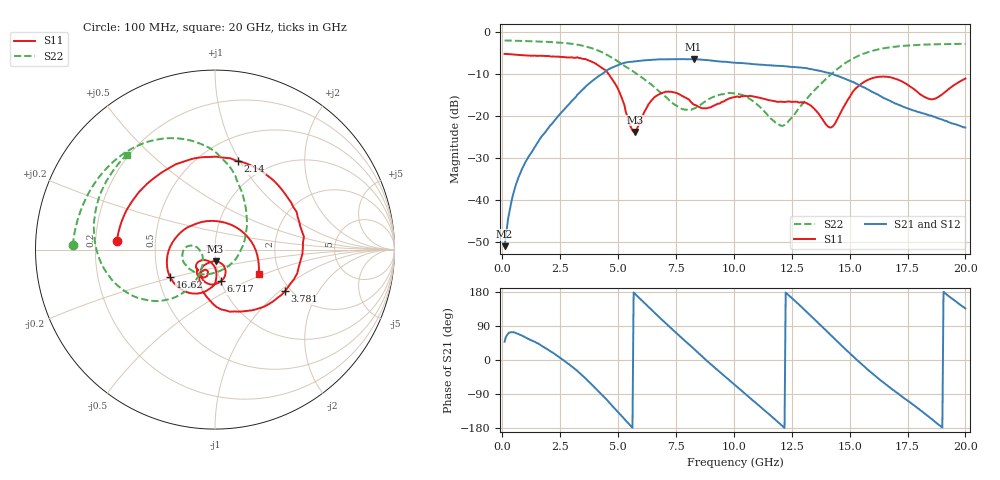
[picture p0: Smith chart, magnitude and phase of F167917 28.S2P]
!  2-Port S-parameters saved by WinCal
! VAR MeasName=S-Parameters (CALIBRATED_DATA) read from VNA (N5242A)
! VAR MeasDate=2016-11-22 9:01:05
! VAR NAME=F167917 28
! VAR FILENAME=F167917 28.S2P
! VAR DATE=2016-11-22 9:01:05
! VAR PHYS_PORTS=1,2
# Hz S DB R 50
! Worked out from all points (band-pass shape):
!   401 points, 100 MHz to 20 GHz, reference 50 ohm
!   highest |S21| = -6.45 dB at 8.259 GHz (marker M1); lowest = -50.9 dB at 100 MHz (marker M2)
!   |S21| within 3 dB of the highest: 4.438 GHz to 13.87 GHz (9.427 GHz wide, 103 % of centre)
!   lowest |S11| = -23.8 dB at 5.722 GHz (marker M3), VSWR 1.14, Z = 49.9 - j6.49 ohm
!   |S11| at or under -10 dB: 4.59 GHz to end of sweep
!   |S22| runs from -22.3 to -2.0 dB; largest |S21 - S12| = 0.0036
!   S11 on the Smith chart (normalised r, x): 100 MHz: 0.29, +0.04; 2.14 GHz: 0.74, +0.98; 3.781 GHz: 1.86, -1.09; 6.717 GHz: 1.01, -0.36; 16.62 GHz: 0.58, -0.19; 20 GHz: 1.56, -0.46
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1e8  -5.22 175.2  -50.91 48.4  -51.07 48.4  -2.03 178.3
7.4675e8  -5.49 144.9  -33.95 67.0  -33.88 66.8  -2.12 167.8
2.13975e9  -5.87 75.5  -21.85 20.6  -21.84 20.3  -2.42 144.5
3.43325e9  -6.33 -6.0  -13.90 -39.7  -13.90 -39.6  -3.23 116.9
3.7815e9  -6.87 -30.8  -12.12 -59.8  -12.10 -59.7  -3.72 108.1
4.82625e9  -11.91 -103.1  -8.27 -126.2  -8.24 -126.4  -6.39 81.3
5.72175e9  -23.76 -87.0  -7.00 175.2  -6.99 175.1  -9.64 61.2
6.71675e9  -14.98 -78.7  -6.53 116.4  -6.53 116.5  -13.88 31.0
6.7665e9  -14.86 -80.7  -6.52 113.6  -6.51 113.6  -14.11 29.0
7.463e9  -14.41 -106.3  -6.49 74.2  -6.46 74.2  -17.35 -10.1
8.259e9  -17.24 -120.5  -6.45 30.2  -6.43 30.2  -18.25 -78.7
9.055e9  -17.73 -107.3  -6.83 -14.0  -6.80 -14.0  -15.59 -128.9
1.005e10  -15.47 -113.1  -7.31 -66.1  -7.29 -66.0  -14.65 -168.3
1.099525e10  -15.52 -126.7  -7.72 -115.5  -7.67 -115.6  -17.19 170.6
1.208975e10  -16.61 -129.6  -8.10 -173.8  -8.05 -173.9  -22.32 -158.7
1.338325e10  -17.80 -142.2  -8.87 112.9  -8.86 113.0  -14.40 -122.0
1.4229e10  -22.60 -111.6  -9.99 63.2  -9.97 63.4  -9.90 -128.0
1.53235e10  -13.14 -97.9  -12.38 -0.2  -12.34 0.1  -5.81 -148.7
1.6617e10  -10.66 -148.4  -16.04 -66.7  -15.93 -66.8  -3.76 -176.2
1.67165e10  -10.74 -152.8  -16.27 -71.5  -16.25 -71.4  -3.68 -178.1
1.8408e10  -15.87 95.8  -19.77 -148.9  -19.70 -149.2  -2.97 154.1
2e10  -11.07 -29.4  -22.72 136.0  -22.56 136.4  -2.84 132.8
